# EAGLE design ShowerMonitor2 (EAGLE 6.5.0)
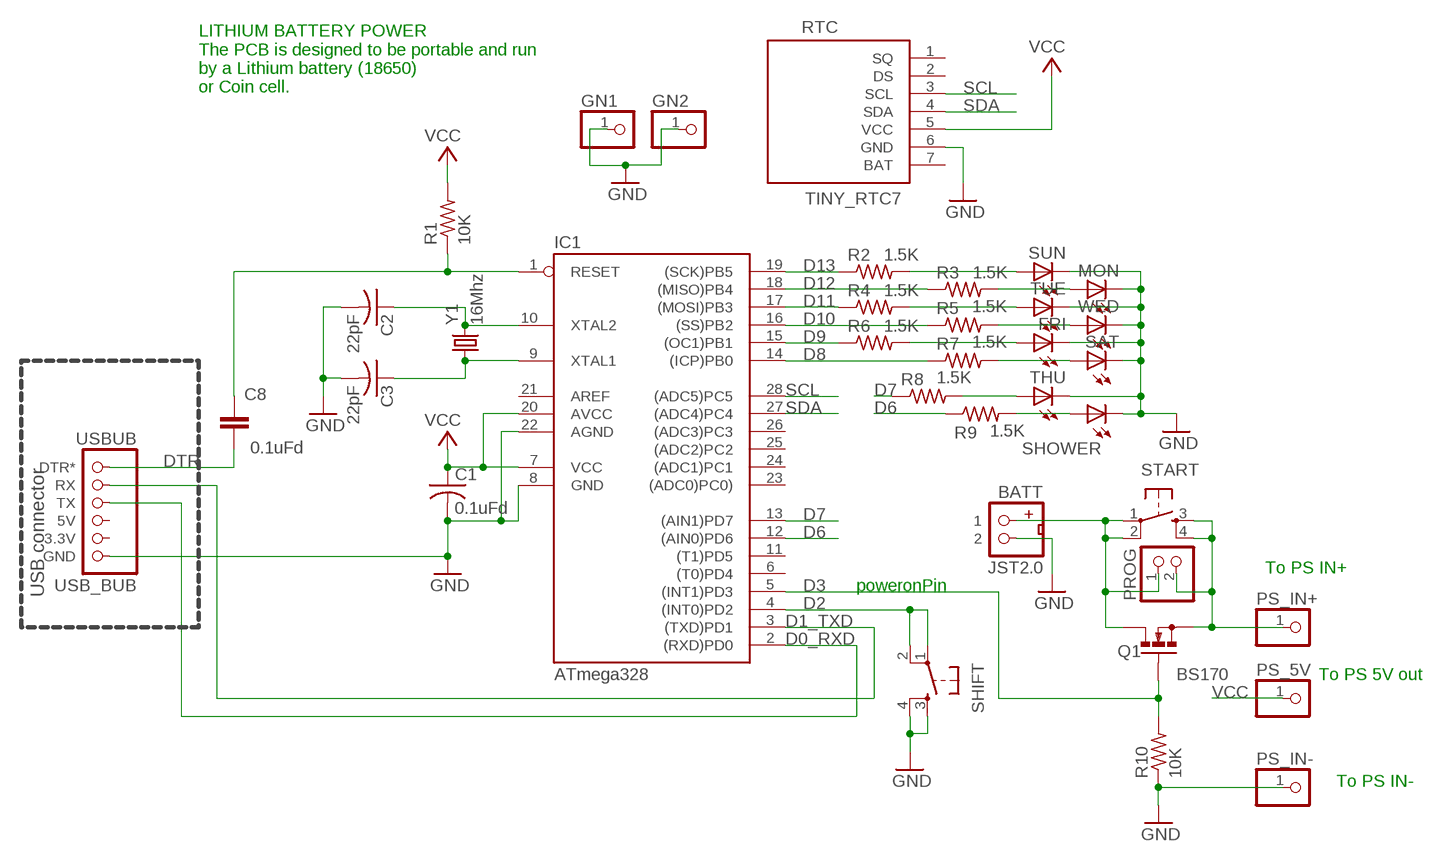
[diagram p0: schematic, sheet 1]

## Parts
BATT  JST2.0  [JST2.0]
C1  0.1uFd  C-US050-024X044  [C050-024X044]
C2  22pF  C-US025-025X050  [C025-025X050]
C3  22pF  C-US025-025X050  [C025-025X050]
C8  0.1uFd  C-EU050-025X075  [C050-025X075]
FRI  LED3MM  [LED3MM]
GN1  PINHD-1X1  [1X01]
GN2  PINHD-1X1  [1X01]
IC1  ATmega328  AT90S4433P  [DIL28-3]
MON  LED3MM  [LED3MM]
PROG  PINHD-1X2/90  [1X02/90]
PS_5V  PINHD-1X1  [1X01]
PS_IN+  PINHD-1X1  [1X01]
PS_IN-  PINHD-1X1  [1X01]
Q1  BS170  [SOT54E]
R1  10K  R-US_0207/7  [0207/7]
R2  1.5K  R-US_0207/2V  [0207/2V]
R3  1.5K  R-US_0207/2V  [0207/2V]
R4  1.5K  R-US_0207/2V  [0207/2V]
R5  1.5K  R-US_0207/2V  [0207/2V]
R6  1.5K  R-US_0207/2V  [0207/2V]
R7  1.5K  R-US_0207/2V  [0207/2V]
R8  1.5K  R-US_0207/2V  [0207/2V]
R9  1.5K  R-US_0207/2V  [0207/2V]
R10  10K  R-US_0207/7  [0207/7]
RTC  TINY_RTC7  [TINY_RTC7]
SAT  LED3MM  [LED3MM]
SHIFT  TAC_SWITCHPTH  [TACTILE-PTH]
SHOWER  LED3MM  [LED3MM]
START  TAC_SWITCHPTH  [TACTILE-PTH]
SUN  LED3MM  [LED3MM]
THU  LED3MM  [LED3MM]
TUE  LED3MM  [LED3MM]
USBUB  USB_BUB  [USB_BUB]
WED  LED3MM  [LED3MM]
Y1  16Mhz  CRYSTALTC38H  [TC38H]

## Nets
D0_RXD: IC1.2((RXD)PD0) USBUB.TX
D1_TXD: IC1.3((TXD)PD1) USBUB.RX
D2: IC1.4((INT0)PD2) SHIFT.1 SHIFT.2
D3: IC1.5((INT1)PD3) Q1.G R10.2
D6: IC1.12((AIN0)PD6) R9.1
D7: IC1.13((AIN1)PD7) R8.1
D8: IC1.14((ICP)PB0) R7.1
D9: IC1.15((OC1)PB1) R6.1
D10: IC1.16((SS)PB2) R5.1
D11: IC1.17((MOSI)PB3) R4.1
D12: IC1.18((MISO)PB4) R3.1
D13: IC1.19((SCK)PB5) R2.1
DTR: C8.1 USBUB.DTR*
GND [power]: BATT.2 C1.2 C2.2 C3.2 FRI.K(C) GN1.1 GN2.1 IC1.8(GND) IC1.22(AGND) MON.K(C) PS_IN-.1 R10.1 RTC.6(GND) SAT.K(C) SHIFT.3 SHIFT.4 SHOWER.K(C) SUN.K(C) THU.K(C) TUE.K(C) USBUB.GND WED.K(C)
N$1: R2.2 SUN.A
N$2: R8.2 THU.A
N$3: MON.A R3.2
N$4: R4.2 TUE.A
N$5: R5.2 WED.A
N$6: C3.1 IC1.9(XTAL1) Y1.1
N$7: C2.1 IC1.10(XTAL2) Y1.2
N$8: FRI.A R6.2
N$9: R7.2 SAT.A
N$11: BATT.1 PROG.1 Q1.D START.1 START.2
N$12: R9.2 SHOWER.A
N$15: PROG.2 PS_IN+.1 Q1.S START.3 START.4
RESET: C8.2 IC1.1(RESET) R1.1
SCL: IC1.28((ADC5)PC5) RTC.3(SCL)
SDA: IC1.27((ADC4)PC4) RTC.4(SDA)
VCC: C1.1 IC1.7(VCC) IC1.20(AVCC) PS_5V.1 R1.2 RTC.5(VCC)
Unconnected: IC1.6((T0)PD4) IC1.11((T1)PD5) IC1.21(AREF) IC1.23((ADC0)PC0)) IC1.24((ADC1)PC1) IC1.25((ADC2)PC2) IC1.26((ADC3)PC3) RTC.1(SQ) RTC.2(DS) RTC.7(BAT) USBUB.3.3V USBUB.5V

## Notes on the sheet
- LITHIUM BATTERY POWER
  The PCB is designed to be portable and run
  by a Lithium battery (18650)
  or Coin cell.
- To PS IN+
- poweronPin
- USB connector
- To PS 5V out
- To PS IN-

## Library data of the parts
BATT = MTS_Custom:JST2.0
C1-C3 = MTS:C-US: CAPACITOR, American symbol
C8 = my-rcl:C-EU: CAPACITOR, European symbol
FRI MON SAT SHOWER SUN THU TUE WED = adafruit:LED: LED
GN1 GN2 PS_5V PS_IN+ PS_IN- = pinhead:PINHD-1X1: PIN HEADER
IC1 = atmel:AT90S4433: MICROCONTROLLER 4 Kbytes FLASH 128 bytes SRAM 256 bytes EEPROM UART 6-channel 10 bit ADC
PROG = pinhead:PINHD-1X2: PIN HEADER
Q1 = transistor-small-signal:BS170: N-CHANNEL MOS FET
R1-R10 = MTS:R-US_: RESISTOR, American symbol
RTC = MTS_Custom:TINY_RTC7
SHIFT START = SparkFun:TAC_SWITCH: Momentary Switch Button commonly used for reset or general input. Spark Fun Electronics SKU : COM-00097
USBUB = MTS:USB_BUB
Y1 = MTS:CRYSTAL: Crystals

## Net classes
0 default: width 0.4 mm, clearance 0.3 mm
1 power: width 0.6 mm, clearance 0.3 mm

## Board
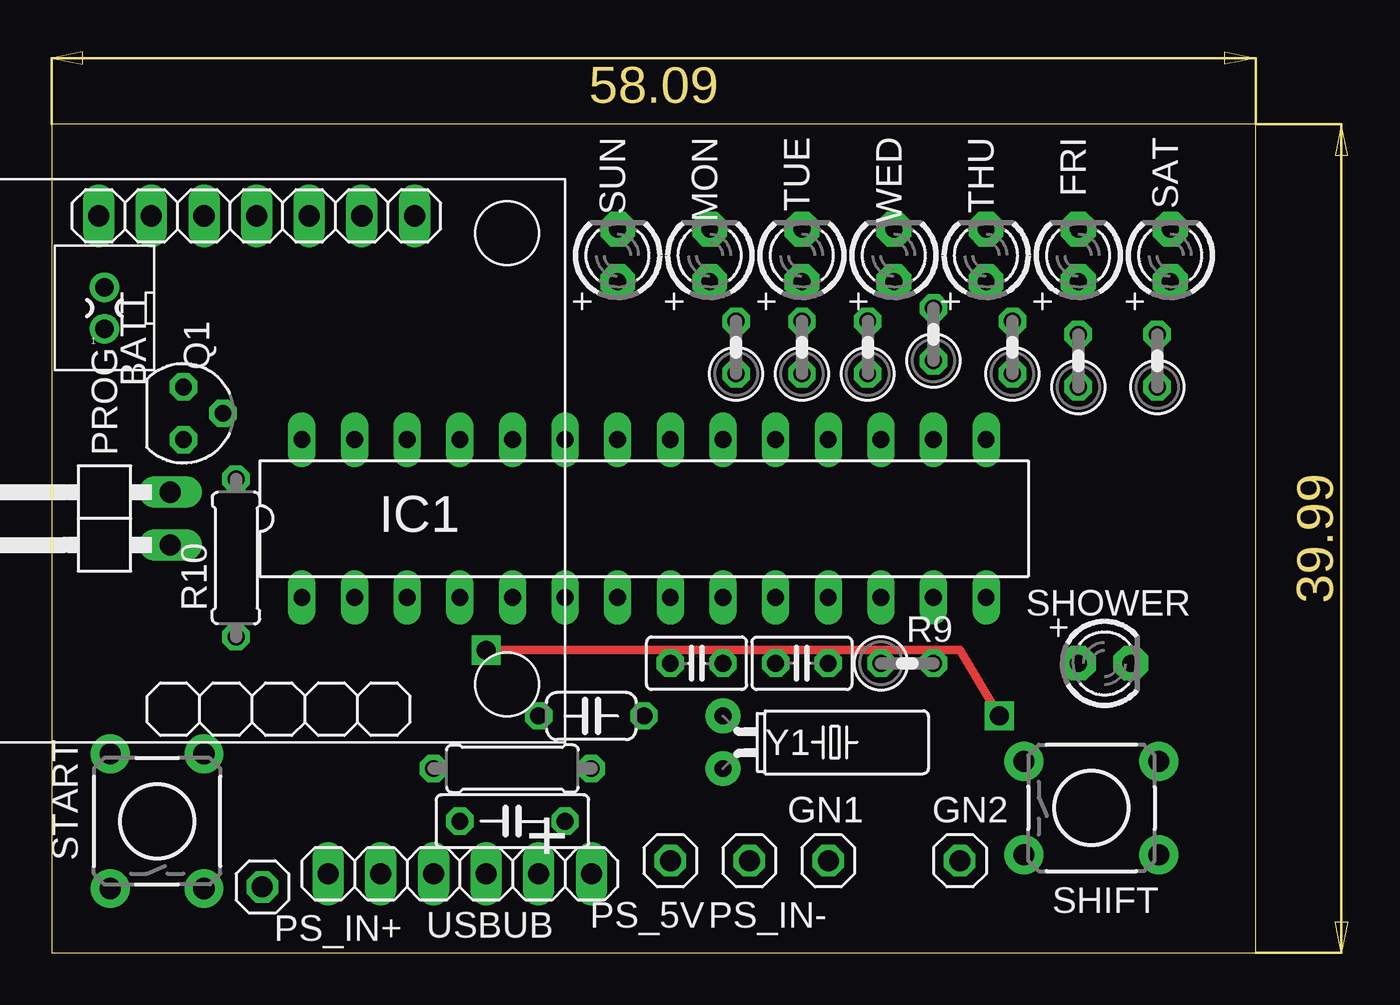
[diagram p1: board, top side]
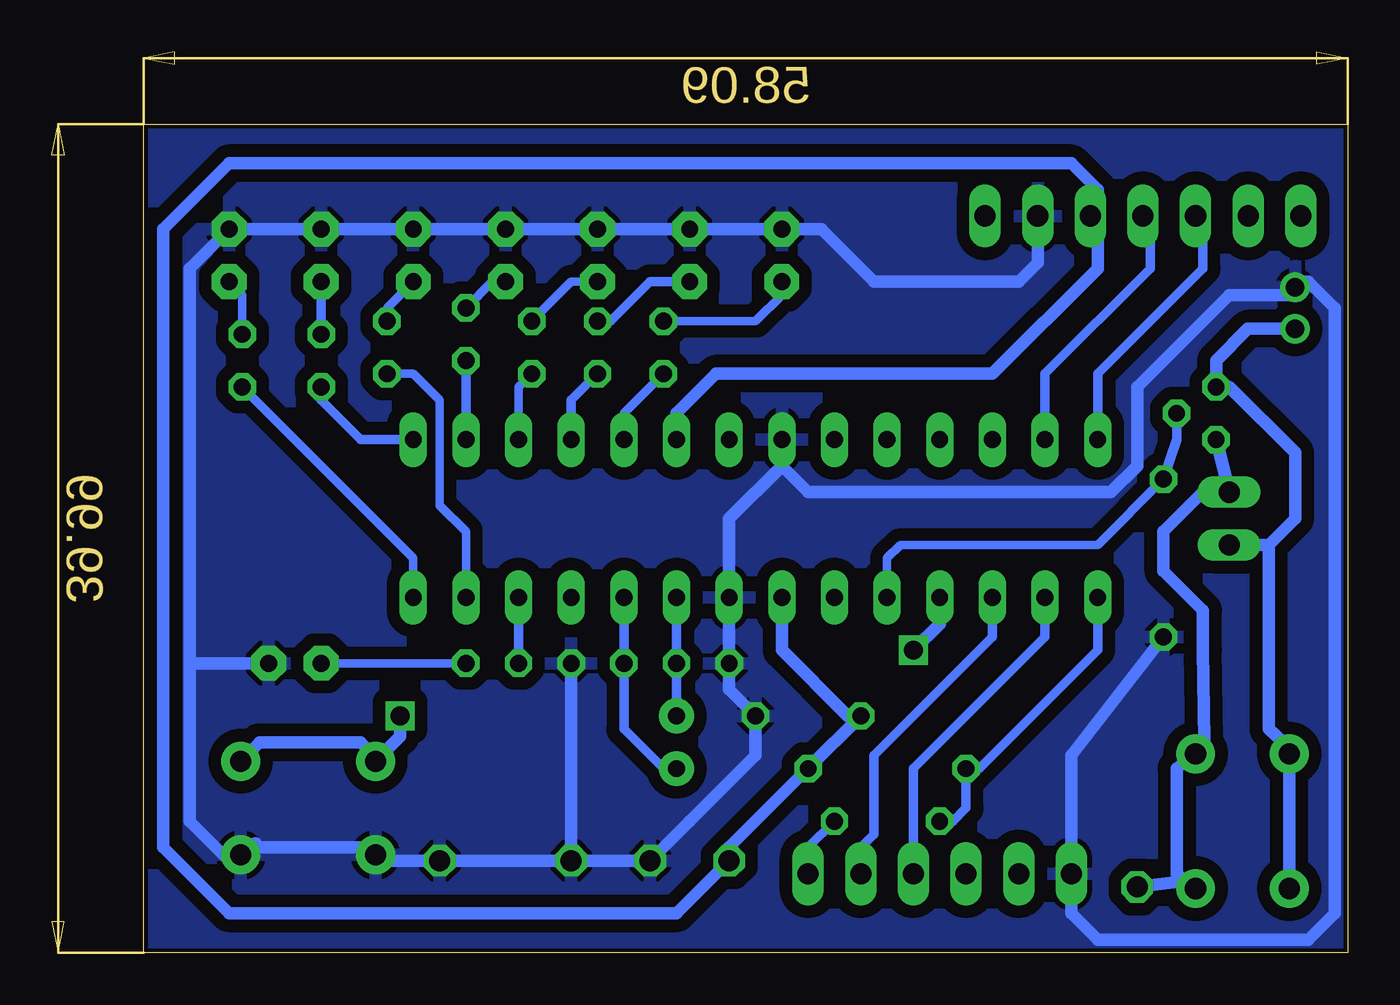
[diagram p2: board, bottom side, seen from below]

Size 62.53 x 43.48 mm. Coordinates in mm from the lower left corner, seen from the top.
Outline: 0,0 58.09,0 58.09,39.99 0,39.99 0,0
Copper layers (1*16): Top 0.035mm / dielectric 1.5mm / Bottom 0.035mm
Design rules "MTS": minimum track width 18mil, minimum drill 12mil, track to track 24mil, track to pad 24mil, pad to pad 6mil, via to via 6mil, smd to smd 0mil, copper to edge 8mil, drill to drill 10mil, minimum pad ring 10mil, minimum via ring 10mil, stop-mask expansion 2mil, vias tented up to drill 25mil, thermal gap 10mil

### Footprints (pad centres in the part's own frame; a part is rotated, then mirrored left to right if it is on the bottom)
JST2.0 = drill 0.9 pad 1.016: 1 0,-1; 2 0,1
C050-024X044 = drill 0.813 octagon: 1 -2.54,0; 2 2.54,0
C025-025X050 = drill 0.813 octagon: 1 -1.27,0; 2 1.27,0
C050-025X075 = drill 0.813 octagon: 1 -2.54,0; 2 2.54,0
LED3MM = drill 0.813 pad 1.676 octagon: A -1.27,0; K 1.27,0
1X01 = drill 1.016 octagon: 1 0,0
DIL28-3 = drill 0.813 long: 1 -16.51,-3.81; 2 -13.97,-3.81; 3 -11.43,-3.81; 4 -8.89,-3.81; 5 -6.35,-3.81; 6 -3.81,-3.81; 7 -1.27,-3.81; 8 1.27,-3.81; 9 3.81,-3.81; 10 6.35,-3.81; 11 8.89,-3.81; 12 11.43,-3.81; 13 13.97,-3.81; 14 16.51,-3.81; 15 16.51,3.81; 16 13.97,3.81; 17 11.43,3.81; 18 8.89,3.81; 19 6.35,3.81; 20 3.81,3.81; 21 1.27,3.81; 22 -1.27,3.81; 23 -3.81,3.81; 24 -6.35,3.81; 25 -8.89,3.81; 26 -11.43,3.81; 27 -13.97,3.81; 28 -16.51,3.81
1X02/90 = drill 1.016 long: 1 -1.27,-3.81; 2 1.27,-3.81
SOT54E = drill 0.813 octagon: D -1.27,0; G 0,1.905; S 1.27,0
0207/7 = drill 0.813 octagon: 1 -3.81,0; 2 3.81,0
0207/2V = drill 0.813 octagon: 1 -1.27,0; 2 1.27,0
TINY_RTC7 = drill 1.016 long: 1 25.4,22.504; 2 25.4,19.964; 3 25.4,17.424; 4 25.4,14.884; 5 25.4,12.344; 6 25.4,9.804; 7 25.4,7.264
TACTILE-PTH = drill 1.016 pad 1.88: 1 -3.251,2.261; 2 3.251,2.261; 3 -3.251,-2.261; 4 3.251,-2.261
USB_BUB = drill 1.016 long: 3.3V -3.81,0; 5V -1.27,0; DTR* 6.35,0; GND -6.35,0; RX 3.81,0; TX 1.27,0
TC38H = drill 0.813 pad 1.676: 1 -1.27,0; 2 1.27,0

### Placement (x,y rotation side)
BATT  2.54,31.11 0 top
C1  26.04,11.43 0 top
C2  36.2,13.97 0 top
C3  31.11,13.97 180 top
C8  22.23,6.35 180 top
FRI  49.53,33.66 90 top
GN1  37.47,4.45 0 top
GN2  43.81,4.45 0 top
IC1  28.57,20.95 0 top
MON  31.75,33.66 90 top
PROG  1.91,20.95 90 top
PS_5V  29.84,4.45 0 top
PS_IN+  10.16,3.17 0 top
PS_IN-  33.66,4.45 0 top
Q1  6.35,26.04 270 top
R1  22.23,8.89 0 top
R2  33.02,29.21 90 top
R3  36.2,29.21 90 top
R4  39.37,29.21 90 top
R5  42.55,29.84 90 top
R6  49.53,28.57 90 top
R7  53.34,28.57 90 top
R8  46.35,29.21 90 top
R9  41.27,13.97 0 top
R10  8.89,19.05 90 top
RTC  24.77,10.16 90 top
SAT  53.98,33.66 90 top
SHIFT  50.16,6.99 0 top
SHOWER  50.8,13.97 0 top
START  5.08,6.35 90 top
SUN  27.3,33.66 90 top
THU  45.09,33.66 90 top
TUE  36.2,33.66 90 top
USBUB  19.68,3.81 0 top
WED  40.64,33.66 90 top
Y1  32.38,10.16 270 top

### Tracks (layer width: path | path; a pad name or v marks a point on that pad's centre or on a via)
D0_RXD
  Bottom 0.457: USBUB.TX 20.95,8.89 14.61,15.24 IC1.2
D1_TXD
  Bottom 0.457: IC1.3 17.14,15.24 22.86,9.53 22.86,5.71 23.5,5.08 USBUB.RX
D2  (via drill 0.9)
  Top 0.406: v20.95,14.61 43.81,14.61 v45.72,11.43
  Bottom 0.61: SHIFT.2 52.5,10.16 47.62,10.16 46.71,9.25 SHIFT.1 45.72,10.44 v45.72,11.43 | IC1.4 19.68,15.88 v20.95,14.61
D3
  Bottom 0.406: R10.2 12.06,19.68 21.59,19.68 22.23,19.05 IC1.5
  Bottom 0.457: R10.2 8.26,24.77 Q1.G
D6
  Bottom 0.457: IC1.12 R9.1
D7
  Bottom 0.406: R8.1 45.09,27.94 43.81,26.67 43.81,21.59 42.55,20.32 IC1.13
D8
  Bottom 0.406: R7.1 45.09,19.05 IC1.14
D9
  Bottom 0.457: IC1.15 47.62,24.77 49.53,26.67 R6.1
D10
  Bottom 0.457: R5.1 IC1.16
D11
  Bottom 0.406: IC1.17 40.01,27.3 R4.1
D12
  Bottom 0.457: IC1.18 37.47,26.67 R3.1
D13
  Bottom 0.406: IC1.19 34.92,26.04 R2.1
DTR
  Bottom 0.457: USBUB.DTR* 26.04,5.08 C8.1
GND
  Bottom 0.6: 53.34,5.08 46.99,5.08 SHIFT.3 46.35,4.45 GN2.1 GN1.1 C2.2 | MON.K TUE.K WED.K | SAT.K 55.88,33.02 55.88,13.97 55.88,8.26 | R10.1 13.34,9.53 USBUB.GND | 27.3,23.5 29.84,20.95 IC1.8 C3.2 29.84,12.7 C1.2 28.57,9.53 31.75,6.35 | 26.04,22.23 27.3,23.5 | 27.3,23.5 IC1.22 | 5.08,31.75 2.54,31.75 BATT.2
  Bottom 0.61: 53.34,5.08 52.7,5.28 SHIFT.4 53.7,4.45 53.98,4.45 55.88,6.35 55.88,8.26 | SHOWER.K 55.88,13.97 | 26.04,22.23 11.43,22.23 10.16,23.5 10.16,27.3 5.71,31.75 5.08,31.75 | USBUB.GND 13.34,1.91 12.06,0.64 1.91,0.64 0.64,1.91 0.64,31.11 1.91,32.38 2.27,32.38 BATT.2 | WED.K THU.K FRI.K SAT.K | MON.K SUN.K 25.4,34.92 22.86,32.38 15.88,32.38 14.96,33.3 RTC.6 | GN1.1 PS_IN-.1 31.75,6.35
  pour Bottom: 0,0 59.05,0 59.05,40.64 0,40.64
N$1
  Bottom 0.406: R2.2 28.57,30.48 27.3,31.75 SUN.A
N$2
  Bottom 0.406: R8.2 46.35,31.11 THU.A
N$3
  Bottom 0.457: R3.2 35.56,30.48 33.66,32.38 MON.A
N$4
  Bottom 0.406: R4.2 37.47,32.38 TUE.A
N$5
  Bottom 0.457: R5.2 41.27,32.38 WED.A
N$6
  Bottom 0.457: IC1.9 C3.1 Y1.1
N$7
  Bottom 0.457: IC1.10 C2.1 34.92,10.79 33.02,8.89 Y1.2
N$8
  Bottom 0.457: FRI.A R6.2
N$9
  Bottom 0.406: R7.2 53.34,31.75 SAT.A
N$11
  Bottom 0.61: 3.81,19.68 3.81,10.79 2.82,9.88 START.2 START.1 | PROG.1 3.81,19.68 | 3.81,19.68 2.54,20.95 2.54,24.13 5.71,27.3 Q1.D 6.35,28.57 4.81,30.11 BATT.1
N$12
  Bottom 0.406: SHOWER.A R9.2
N$15
  Bottom 0.61: PS_IN+.1 7.98,3.45 START.3 8.26,3.81 8.26,8.89 START.4 6.91,10.24 6.99,14.61 6.99,16.51 8.89,18.41 8.89,20.32 6.99,22.23 PROG.2 Q1.S
RESET
  Bottom 0.457: C8.2 19.05,6.35 18.41,6.99 R1.1 17.78,8.89 12.06,14.61 IC1.1
SCL
  Bottom 0.457: IC1.28 12.06,27.94 6.99,33.02 6.99,34.92 RTC.3
SDA
  Bottom 0.457: IC1.27 14.61,27.94 9.53,33.02 9.53,34.92 RTC.4
VCC
  Bottom 0.61: 12.06,36.83 12.06,33.02 17.14,27.94 30.48,27.94 32.38,26.04 IC1.20 | 12.06,36.83 13.34,38.1 53.98,38.1 57.15,34.92 57.15,5.08 53.98,1.91 32.38,1.91 PS_5V.1 29.84,5.08 R1.2 C1.1 24.13,11.43 27.3,14.61 IC1.7 | 12.06,36.83 RTC.5

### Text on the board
tNames: +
